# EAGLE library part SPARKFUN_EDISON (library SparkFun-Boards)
SparkFun Edison The Intel® Edison is an ultra small computing platform that will change the way you look at embedded electronics. Each Edison packs a huge amount of tech goodies into a tiny package while still providing the same robust strength of your go-to single board computer. Powered by the Intel® Atom™ SoC dual-core CPU and including an integrated WiFi, Bluetooth LE, and a 70-pin connector to attach a veritable slew of shield-like “Blocks” which can be stacked on top of each other. This device includes footprints for the Edison module itself, as well as the basic board outline used for our Edison blocks. SparkFun Products: Intel Edison SparkFun Console Block SparkFun GPIO Block SparkFun Battery Block SparkFun Base Block SparkFun 9DOF Block SparkFun OLED Block SparkFun Dual H-Bridge Block SparkFun microSD Block SparkFun ADC Block SparkFun I2C Block SparkFun Arduino Block SparkFun Power Block SparkFun PWM Block SparkFun Raspberry Pi Block SparkFun UART Block
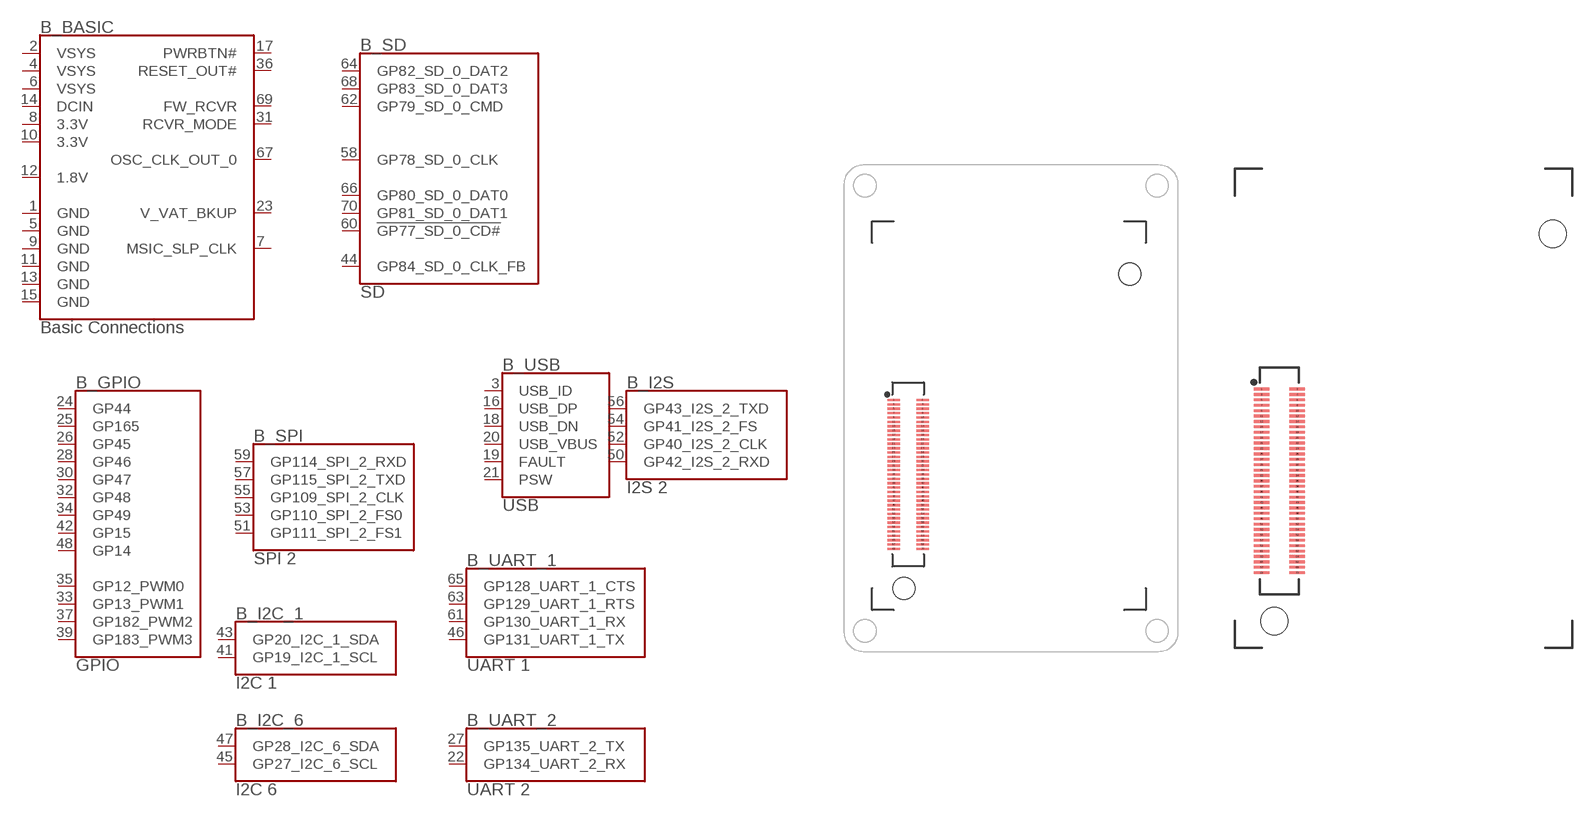
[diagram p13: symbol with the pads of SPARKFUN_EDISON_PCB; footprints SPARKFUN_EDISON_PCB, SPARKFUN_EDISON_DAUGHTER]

Designator prefix B; gates _BASIC=EDISON_CONNECTOR_BASE _GPIO=EDISON_CONNECTOR_GPIO _I2C_1=EDISON_CONNECTOR_I2C_1 _I2C_6=EDISON_CONNECTOR_I2C_6 _I2S=EDISON_CONNECTOR_I2S_2 _SD=EDISON_CONNECTOR_SD _SPI=EDISON_CONNECTOR_SPI_2 _UART_1=EDISON_CONNECTOR_UART_1 _UART_2=EDISON_CONNECTOR_UART_2 _USB=EDISON_CONNECTOR_USB

## SPARKFUN_EDISONPCB  [SPARKFUN_EDISON_PCB]
1  _BASIC:GND  pwr
2  _BASIC:VSYS  pwr
3  _USB:USB_ID
4  _BASIC:VSYS  pwr
5  _BASIC:GND  pwr
6  _BASIC:VSYS  pwr
7  _BASIC:MSIC_SLP_CLK
8  _BASIC:3.3V  pwr
9  _BASIC:GND  pwr
10  _BASIC:3.3V  pwr
11  _BASIC:GND  pwr
12  _BASIC:1.8V  pwr
13  _BASIC:GND  pwr
14  _BASIC:DCIN  pwr
15  _BASIC:GND  pwr
16  _USB:USB_DP
17  _BASIC:PWRBTN#
18  _USB:USB_DN
19  _USB:FAULT
20  _USB:USB_VBUS
21  _USB:PSW
22  _UART_2:GP134_UART_2_RX
23  _BASIC:V_VAT_BKUP  pwr
24  _GPIO:GP44
25  _GPIO:GP165
26  _GPIO:GP45
27  _UART_2:GP135_UART_2_TX
28  _GPIO:GP46
30  _GPIO:GP47
31  _BASIC:RCVR_MODE
32  _GPIO:GP48
33  _GPIO:GP13_PWM1
34  _GPIO:GP49
35  _GPIO:GP12_PWM0
36  _BASIC:RESET_OUT#
37  _GPIO:GP182_PWM2
39  _GPIO:GP183_PWM3
41  _I2C_1:GP19_I2C_1_SCL
42  _GPIO:GP15
43  _I2C_1:GP20_I2C_1_SDA
44  _SD:GP84_SD_0_CLK_FB
45  _I2C_6:GP27_I2C_6_SCL
46  _UART_1:GP131_UART_1_TX
47  _I2C_6:GP28_I2C_6_SDA
48  _GPIO:GP14
50  _I2S:GP42_I2S_2_RXD
51  _SPI:GP111_SPI_2_FS1
52  _I2S:GP40_I2S_2_CLK
53  _SPI:GP110_SPI_2_FS0
54  _I2S:GP41_I2S_2_FS
55  _SPI:GP109_SPI_2_CLK
56  _I2S:GP43_I2S_2_TXD
57  _SPI:GP115_SPI_2_TXD
58  _SD:GP78_SD_0_CLK
59  _SPI:GP114_SPI_2_RXD
60  _SD:!GP77_SD_0_CD#
61  _UART_1:GP130_UART_1_RX
62  _SD:GP79_SD_0_CMD
63  _UART_1:GP129_UART_1_RTS
64  _SD:GP82_SD_0_DAT2
65  _UART_1:GP128_UART_1_CTS
66  _SD:GP80_SD_0_DAT0
67  _BASIC:OSC_CLK_OUT_0
68  _SD:GP83_SD_0_DAT3
69  _BASIC:FW_RCVR
70  _SD:GP81_SD_0_DAT1

## SPARKFUN_EDISON  [SPARKFUN_EDISON_DAUGHTER]
Pads as for SPARKFUN_EDISON_PCB

## Footprint SPARKFUN_EDISON_PCB (pad centres in mm)
SparkFun Edison PCB Footprint for Edison PCBs (view that mates with Edison SBC). Specifications: Pin count:11 Area:1.20 x 1.75 inch Example device(s): SparkFun Edison
smd 1.14 x 0.2: 1 -10.72,1.39; 2 -8.08,1.39; 3 -10.72,0.99; 4 -8.08,0.99; 5 -10.72,0.59; 6 -8.08,0.59; 7 -10.72,0.19; 8 -8.08,0.19; 9 -10.72,-0.21; 10 -8.08,-0.21; 11 -10.72,-0.61; 12 -8.08,-0.61; 13 -10.72,-1.01; 14 -8.08,-1.01; 15 -10.72,-1.41; 16 -8.08,-1.41; 17 -10.72,-1.81; 18 -8.08,-1.81; 19 -10.72,-2.21; 20 -8.08,-2.21; 21 -10.72,-2.61; 22 -8.08,-2.61; 23 -10.72,-3.01; 24 -8.08,-3.01; 25 -10.72,-3.41; 26 -8.08,-3.41; 27 -10.72,-3.81; 28 -8.08,-3.81; 29 -10.72,-4.21; 30 -8.08,-4.21; 31 -10.72,-4.61; 32 -8.08,-4.61; 33 -10.72,-5.01; 34 -8.08,-5.01; 35 -10.72,-5.41; 36 -8.08,-5.41; 37 -10.72,-5.81; 38 -8.08,-5.81; 39 -10.72,-6.21; 40 -8.08,-6.21; 41 -10.72,-6.61; 42 -8.08,-6.61; 43 -10.72,-7.01; 44 -8.08,-7.01; 45 -10.72,-7.41; 46 -8.08,-7.41; 47 -10.72,-7.81; 48 -8.08,-7.81; 49 -10.72,-8.21; 50 -8.08,-8.21; 51 -10.72,-8.61; 52 -8.08,-8.61; 53 -10.72,-9.01; 54 -8.08,-9.01; 55 -10.72,-9.41; 56 -8.08,-9.41; 57 -10.72,-9.81; 58 -8.08,-9.81; 59 -10.72,-10.21; 60 -8.08,-10.21; 61 -10.72,-10.61; 62 -8.08,-10.61; 63 -10.72,-11.01; 64 -8.08,-11.01; 65 -10.72,-11.41; 66 -8.08,-11.41; 67 -10.72,-11.81; 68 -8.08,-11.81; 69 -10.72,-12.21; 70 -8.08,-12.21
hole 2 at 10.83,12.89
hole 2 at -9.77,-15.8

## Footprint SPARKFUN_EDISON_DAUGHTER (pad centres in mm)
SparkFun Edison Daughter Footprint for mating with Edison SBC. Specifications: Pin count:11 Area: 0.98 x 1.4 inch Example device(s): SparkFun Edison
smd 1.14 x 0.2: 1 -11.99,1.39; 2 -9.35,1.39; 3 -11.99,0.99; 4 -9.35,0.99; 5 -11.99,0.59; 6 -9.35,0.59; 7 -11.99,0.19; 8 -9.35,0.19; 9 -11.99,-0.21; 10 -9.35,-0.21; 11 -11.99,-0.61; 12 -9.35,-0.61; 13 -11.99,-1.01; 14 -9.35,-1.01; 15 -11.99,-1.41; 16 -9.35,-1.41; 17 -11.99,-1.81; 18 -9.35,-1.81; 19 -11.99,-2.21; 20 -9.35,-2.21; 21 -11.99,-2.61; 22 -9.35,-2.61; 23 -11.99,-3.01; 24 -9.35,-3.01; 25 -11.99,-3.41; 26 -9.35,-3.41; 27 -11.99,-3.81; 28 -9.35,-3.81; 29 -11.99,-4.21; 30 -9.35,-4.21; 31 -11.99,-4.61; 32 -9.35,-4.61; 33 -11.99,-5.01; 34 -9.35,-5.01; 35 -11.99,-5.41; 36 -9.35,-5.41; 37 -11.99,-5.81; 38 -9.35,-5.81; 39 -11.99,-6.21; 40 -9.35,-6.21; 41 -11.99,-6.61; 42 -9.35,-6.61; 43 -11.99,-7.01; 44 -9.35,-7.01; 45 -11.99,-7.41; 46 -9.35,-7.41; 47 -11.99,-7.81; 48 -9.35,-7.81; 49 -11.99,-8.21; 50 -9.35,-8.21; 51 -11.99,-8.61; 52 -9.35,-8.61; 53 -11.99,-9.01; 54 -9.35,-9.01; 55 -11.99,-9.41; 56 -9.35,-9.41; 57 -11.99,-9.81; 58 -9.35,-9.81; 59 -11.99,-10.21; 60 -9.35,-10.21; 61 -11.99,-10.61; 62 -9.35,-10.61; 63 -11.99,-11.01; 64 -9.35,-11.01; 65 -11.99,-11.41; 66 -9.35,-11.41; 67 -11.99,-11.81; 68 -9.35,-11.81; 69 -11.99,-12.21; 70 -9.35,-12.21
hole 2 at 9.56,12.89
hole 2 at -11.04,-15.8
